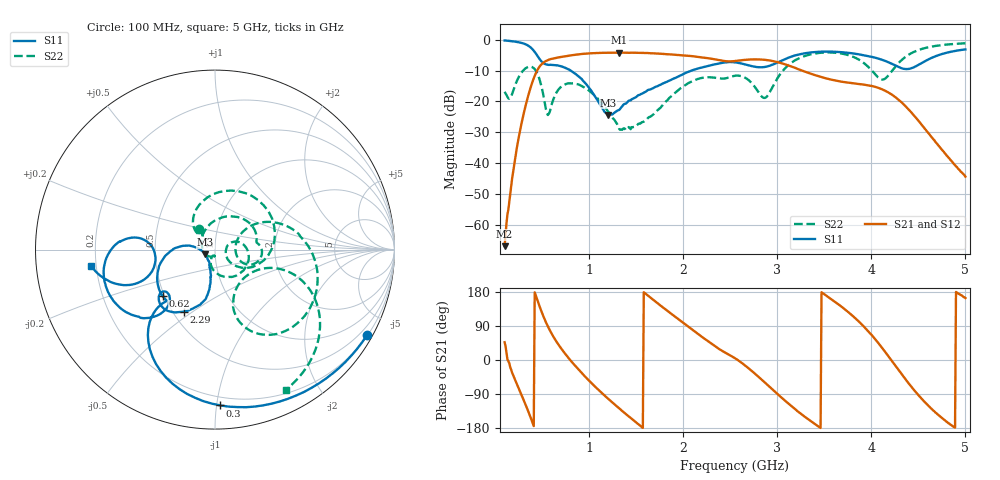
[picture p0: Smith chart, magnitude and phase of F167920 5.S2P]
!  2-Port S-parameters saved by WinCal
! VAR MeasName=S-Parameters (CALIBRATED_DATA) read from VNA (N5242A)
! VAR MeasDate=2016-11-22 9:53:45
! VAR NAME=F167920 5
! VAR FILENAME=F167920 5.S2P
! VAR DATE=2016-11-22 9:53:45
! VAR PHYS_PORTS=1,2
# Hz S DB R 50
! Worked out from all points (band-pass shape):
!   491 points, 100 MHz to 5 GHz, reference 50 ohm
!   highest |S21| = -4.17 dB at 1.32 GHz (marker M1); lowest = -66.8 dB at 100 MHz (marker M2)
!   |S21| within 3 dB of the highest: 524.1 MHz to 2.989 GHz (2.465 GHz wide, 140 % of centre)
!   lowest |S11| = -24.3 dB at 1.2 GHz (marker M3), VSWR 1.13, Z = 44.7 - j2.35 ohm
!   |S11| at or under -10 dB: 802.5 MHz to 2.087 GHz (1.284 GHz wide, 88.9 % of centre)
!   |S22| runs from -29.3 to -1.2 dB; largest |S21 - S12| = 0.002
!   S11 on the Smith chart (normalised r, x): 100 MHz: 0.22, -3.82; 300 MHz: 0.14, -1.02; 620 MHz: 0.49, -0.30; 2.29 GHz: 0.57, -0.46; 5 GHz: 0.18, -0.06
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1e8  -0.25 -29.3  -66.83 46.9  -65.11 39.5  -16.87 128.6
2e8  -0.58 -58.0  -40.85 -45.5  -40.83 -45.5  -15.77 134.9
3e8  -1.22 -88.1  -24.30 -104.1  -24.30 -103.9  -9.89 86.5
4.6e8  -5.74 -133.2  -9.24 149.9  -9.23 149.9  -11.83 -18.3
5.6e8  -8.13 -133.7  -6.62 88.7  -6.61 88.7  -24.37 -7.6
6.2e8  -8.17 -138.2  -6.05 61.0  -6.05 61.0  -19.16 23.0
7.7e8  -9.47 -160.2  -5.24 8.3  -5.23 8.3  -14.17 -16.7
9.2e8  -12.71 179.0  -4.61 -34.2  -4.61 -34.2  -14.99 -58.9
1.2e9  -24.33 -154.5  -4.23 -102.2  -4.23 -102.1  -23.27 -109.8
1.32e9  -22.72 -117.3  -4.17 -127.8  -4.16 -127.8  -28.97 -109.2
1.53e9  -17.90 -101.9  -4.25 -171.1  -4.25 -171.1  -27.15 -108.8
1.74e9  -14.80 -98.0  -4.52 147.3  -4.52 147.3  -22.47 165.5
2.01e9  -10.96 -101.0  -5.08 96.0  -5.07 96.0  -14.94 79.8
2.29e9  -8.28 -116.5  -6.11 44.6  -6.10 44.5  -12.18 23.1
2.55e9  -7.33 -135.5  -6.90 4.7  -6.89 4.6  -11.68 -0.4
2.87e9  -8.82 -134.4  -6.53 -60.0  -6.52 -60.1  -18.83 5.2
3.11e9  -5.93 -132.3  -8.25 -113.3  -8.23 -113.5  -8.45 23.2
3.37e9  -4.08 -149.9  -11.16 -163.7  -11.13 -164.0  -4.64 -13.1
3.77e9  -4.30 -175.2  -13.97 123.2  -13.97 123.0  -5.13 -59.0
4.19e9  -7.41 171.3  -17.25 7.1  -17.25 6.8  -11.24 -23.6
4.51e9  -7.98 -158.4  -26.59 -95.4  -26.62 -95.7  -3.25 -32.2
5e9  -3.15 -172.4  -44.33 163.5  -44.22 163.9  -1.15 -63.3
